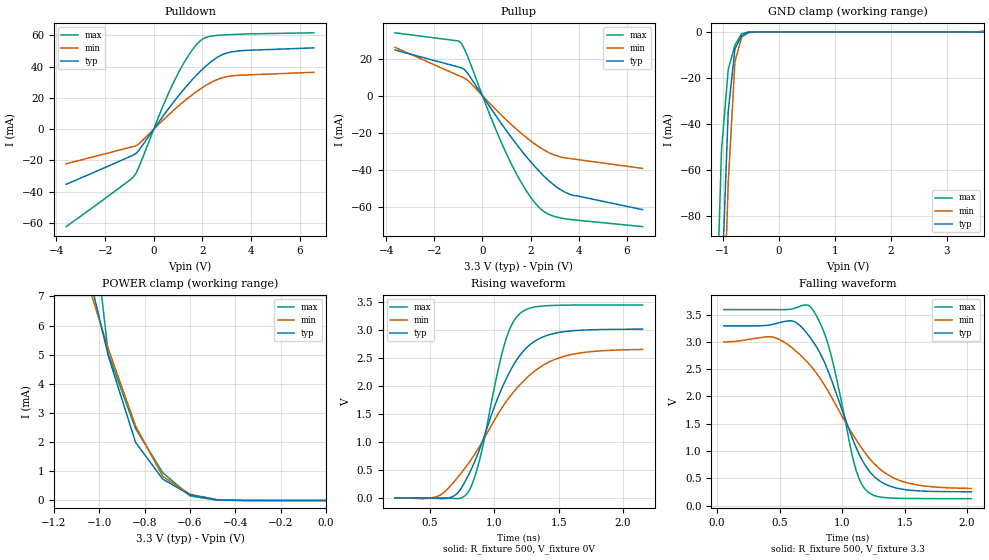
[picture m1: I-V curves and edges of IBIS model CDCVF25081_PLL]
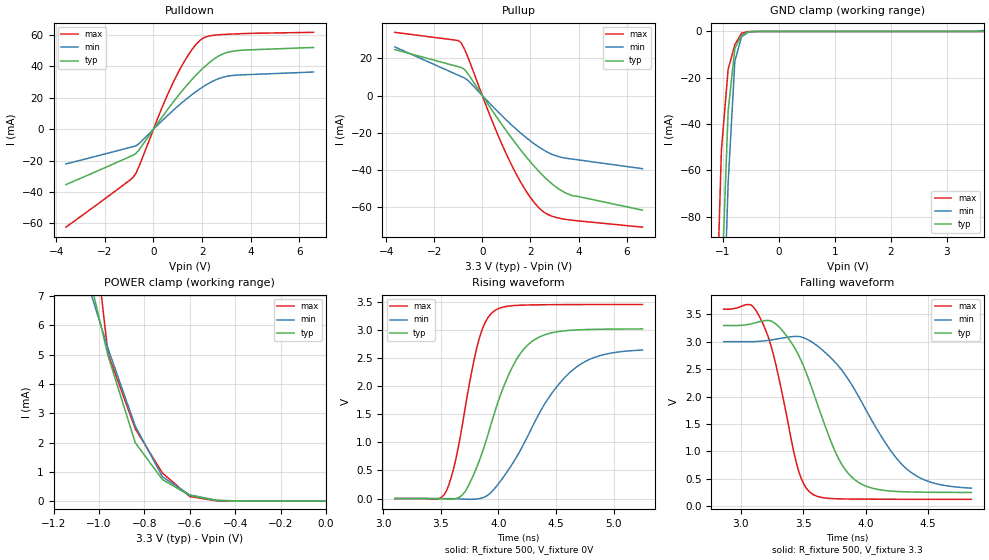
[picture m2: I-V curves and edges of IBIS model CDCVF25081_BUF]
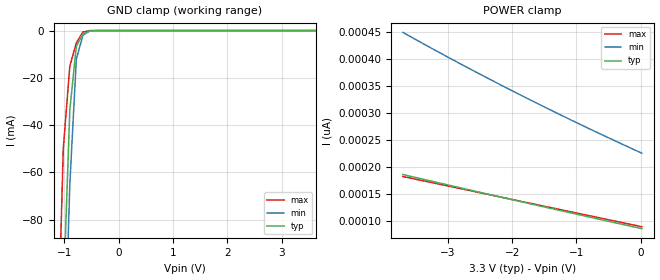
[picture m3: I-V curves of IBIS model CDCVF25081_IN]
[IBIS Ver]   3.2
[File Name]   cvf25081_03.ibs  | DEVICES: CDCVF25081PW
[File Rev]   0.3
[Date]   11/15/2002
[Source]   File originated at Texas Instruments
[Notes]   The following information corresponds to the
|   CDCVF25081 output buffers and input ESD circuits.
|Revision log: 0.1, 11/12/2002  initial release.
|   0.2, 11/15/2002  DC/AC correlation CDCVF25081
|   0.3, 11/22/2002  added model spec parameter
| Simulation hints.
| In PLL-MODE the Vt tables are normalized to have them switching all at the
| same time across TYP/MIN/MAX to reflect the virtual independency on split,
| VDD and temperature due to active phase controll in PLL-MODE.
| However there is a positive offset, since real phase relation in PLL_MODE
| would require negative relation to input signal which can not be simulated
| within IBIS models!
| In simple buffer mode the model works as a buffer and the VT plots represent
| the buffer switching characteristics starting at Vmeas for input signal, which
| initiates the buffer to toggle. If the lead-in delay is unwanted, equally
| substract exact same amount of time from rising AND falling waveforms !
[Disclaimer]
|This information is for modeling purposes only
|and is not guaranteed.
|Property of Texas Instruments Incorporated unauthorized reproduction
|and/or distribution is strictly prohibited.
|This product is protected under copyright law and trade
|secret law as an unpublished work.  Created  1998.
|(C) Copyright 1998 Texas Instruments Incorporated.
|All rights reserved.
|These commodities are under U.S. Government distribution
|license control. As such, they are not to be re-exported
|without prior approval of the U.S. Department of Commerce.
|Please be aware that in the absence of a written agreement
|to the contrary, Texas Instruments ("TI") assumes no
|liability for:  (1) the accuracy of the IBIS Models provided
|to your company;  (2) the proper functioning of these Models
|in your design system or for any resulting applications;
|or (3) infringement of patents, copyrights or intellectual
|property rights resulting from your use of these models.
|TI provides IBIS Models as a service to our customers
|and therefore reserves the right to limit distribution
|of the Models.
|CDCVF25081 IBIS I/O Model
|Mixed Signal Products, Texas Instruments
[Component]   CDCVF25081PW   | 16 Pin TSSOP package
[Manufacturer] Texas Instruments
[Package]
|   typ   min   max
R_pkg   0.0450710   0.0376501   0.0513656
L_pkg   2.5907775n   2.44687n   3.07983n
C_pkg   0.1415751p   0.0907328p   0.270926p
[Pin]   signal_name   model_name   R_pin   L_pin   C_pin
 1   CLK   CDCVF25081_IN   0.0397681   3.07983n   0.270926p
 2   1Y0   CDCVF25081_OUT   0.0376501   2.45757n   0.138771p
 3   1Y1   CDCVF25081_OUT   0.0512415   2.51196n   0.115722p
 4   VDD   POWER   0.0513168   2.44723n   0.090733p
 5   GND   GND   0.0513659   2.44724n   0.097386p
 6   2Y0   CDCVF25081_OUT   0.0512883   2.51196n   0.115722p
 7   2Y1   CDCVF25081_OUT   0.0376511   2.45777n   0.138759p
 8   S2   CDCVF25081_CTRLIN   0.0397673   3.03973n   0.270941p
 9   S1   CDCVF25081_CTRLIN   0.0394705   2.83153n   0.216335p
10   2Y2   CDCVF25081_OUT   0.0384835   2.45963n   0.142304p
11   2Y3   CDCVF25081_OUT   0.0512411   2.51159n   0.115740p
12   GND   GND   0.0513654   2.44687n   0.090831p
13   VDD   POWER   0.0513656   2.44687n   0.090825p
14   1Y2   CDCVF25081_OUT   0.0512413   2.51157n   0.115741p
15   1Y3   CDCVF25081_OUT   0.0384826   2.45948n   0.142306p
16   FBIN   CDCVF25081_IN   0.0394374   2.83161n   0.216310p
[Model Selector]   CDCVF25081_OUT
CDCVF25081_BUF for SIMPLE_BUFFER_MODE
CDCVF25081_PLL for PLL_MODE
| Models and submodels in the file (4): CDCVF25081_PLL (Output), CDCVF25081_BUF (Output), CDCVF25081_IN (Input), CDCVF25081_CTRLIN (Input)
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|   Model CDCVF25081_PLL
[Model]   CDCVF25081_PLL
Model_type   Output
Polarity   Non-Inverting
Enable   Active-High
Vmeas = 1.5V
Cref = 15pF
Rref = 500
Vref = 1.65V
|   variable   typ   min   max
C_comp   2.8pF   NA   NA
[Model Spec]
|  subparameter   typ   min   max
Vmeas   1.65V   1.50V   1.80V
|   variable   typ   min   max
[Temperature Range]   40   85   -40
[Voltage range]   3.3   3.0   3.6
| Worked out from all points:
|   slope of the pulldown table from 0 to 0.495 V, typ, clamps not added: 46.1 ohm
|   slope of the pullup table from 0 to 0.495 V, typ, clamps not added: 51.6 ohm
|   GND clamp passes 1 mA (typ) near -0.61 V on its own axis
|   POWER clamp passes 1 mA (typ) near -0.75 V on its own axis
|   rising waveform, R_fixture 500, V_fixture 0V: 20-80 % time 320ps typ, 470ps min, 194ps max; typ from 0 V to 3.02 V
|   falling waveform, R_fixture 500, V_fixture 3.3: 20-80 % time 307ps typ, 440ps min, 196ps max; typ from 3.3 V to 0.252 V
[Pullup]
|   40C:3.3V:nominal   85C:3.0V:weak   -40C:3.6V:strong
|  Voltage   I(typ)   I(min)   I(max)
-3.64V    24.7mA     26.12mA    33.95mA
-1V       15.51mA    10.93mA    29.56mA
-880mV    15.09mA    10.23mA    28.31mA
-640mV    12.45mA    8.62mA     21.96mA
440mV     -8.541mA   -5.947mA   -14.63mA
1.16V     -21.74mA   -15.05mA   -35.71mA
1.88V     -33.69mA   -23.11mA   -52.38mA
2.24V     -39.05mA   -26.59mA   -58.61mA
2.48V     -42.32mA   -28.63mA   -61.7mA
3.08V     -49.16mA   -32.29mA   -65.37mA
3.66V     -53.25mA   -33.88mA   -66.69mA
6.66V     -61.41mA   -39.18mA   -70.55mA
[Pulldown]
|   40C:3.3V:nominal   85C:3.0V:weak   -40C:3.6V:strong
|  Voltage   I(typ)   I(min)   I(max)
-3.6V     -35.29mA   -22.13mA   -62.34mA
-840mV    -16.57mA   -11.08mA   -30.65mA
-600mV    -13.26mA   -9.226mA   -23.82mA
340mV     7.461mA    5.189mA    13.35mA
820mV     17.44mA    12.14mA    30.1mA
1.3V      26.65mA    18.55mA    44.02mA
1.66V     32.94mA    22.91mA    52.28mA
1.9V      36.78mA    25.56mA    56.37mA
2.14V     40.29mA    27.97mA    58.65mA
2.62V     46.02mA    31.8mA     59.99mA
3.1V      49.13mA    33.84mA    60.45mA
6.58V     52.01mA    36.39mA    61.64mA
[GND Clamp]
|   40C:3.3V:nominal   85C:3.0V:weak   -40C:3.6V:strong
|  Voltage   I(typ)   I(min)   I(max)
-3.66V    -2.664A    -2.705A    -2.597A
-1.26V    -322.6mA   -368.2mA   -247.4mA
-1.02V    -113.4mA   -156.1mA   -51.21mA
-900mV    -34.44mA   -65.67mA   -16.35mA
-780mV    -7.275mA   -12.8mA    -5.698mA
-660mV    -1.683mA   -2.274mA   -709.9uA
-540mV    -157.1uA   -304.4uA   -20.32uA
-420mV    -6.863uA   -22.34uA   -162nA
3.42V     391.2pA    8.031uA    123.3pA
3.66V     873.2nA    432.9uA    136.7pA
[POWER Clamp]
|   40C:3.3V:nominal   85C:3.0V:weak  -40C:3.6V:strong
|  Voltage   I(typ)   I(min)   I(max)
-3.6V     107mA      79mA       290mA
-1.08V    8.909mA    8.202mA    13.19mA
-960mV    4.96mA     5.207mA    5.035mA
-840mV    1.996mA    2.561mA    2.466mA
-720mV    733.3uA    827.9uA    954.8uA
-600mV    191.2uA    212.2uA    157.3uA
-480mV    19.67uA    29.3uA     7.993uA
0V        126.6pA    280.9pA    133.2pA
[ramp]
| variable   typ   min   max
dV/dt_r   1.8115/3.2020E-10   1.5957/4.7143E-10   2.0668/1.9311E-10
dV/dt_f   1.8292/3.0774E-10   1.6162/4.4162E-10   2.0805/1.9637E-10
[Rising Waveform]
R_fixture = 500
V_fixture = 0V
|   40C:3.3V:nominal   85C:3.0V:weak   -40C:3.6V:strong
|   Time   V(typ)   V(min)   V(max)
231ps     0V         100uV      0V
570.5ps   -10.8mV    38.9mV     100uV
690.5ps   38.7mV     292.3mV    -9.4mV
790.5ps   363.5mV    585.1mV    75.9mV
890.5ps   889.4mV    936.1mV    708.3mV
1.091ns   2.116V     1.713V     2.828V
1.211ns   2.58V      2.048V     3.314V
1.351ns   2.846V     2.328V     3.422V
1.551ns   2.972V     2.534V     3.443V
2.151ns   3.015V     2.652V     3.447V
[Falling Waveform]
R_fixture = 500
V_fixture = 3.3
V_fixture_min = 3.0
V_fixture_max = 3.6
|   40C:3.3V:nominal   85C:3.0V:weak -40C:3.6V:strong
|   Time   V(typ)   V(min)   V(max)
54ps      3.296V     3.001V     3.593V
454ps     3.327V     3.085V     3.593V
614ps     3.377V     2.865V     3.613V
754ps     3.053V     2.549V     3.627V
894ps     2.432V     2.074V     2.912V
1.114ns   1.055V     1.202V     634mV
1.214ns   642.4mV    877.8mV    236mV
1.334ns   405.6mV    613.4mV    148.1mV
1.494ns   295.8mV    434.6mV    131.6mV
2.034ns   252.4mV    314.8mV    126.1mV
|   Model CDCVF25081_BUF
[Model]   CDCVF25081_BUF
Model_type   Output
Polarity   Non-Inverting
Enable   Active-High
Vmeas = 1.5V
Cref = 15pF
Rref = 500
Vref = 1.65V
|   variable   typ   min   max
C_comp   2.8pF   NA   NA
[Model Spec]
|  subparameter   typ   min   max
Vmeas   1.65V   1.50V   1.80V
|   variable   typ   min   max
[Temperature Range]   40   85   -40
[Voltage range]   3.3   3.0   3.6
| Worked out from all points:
|   slope of the pulldown table from 0 to 0.495 V, typ, clamps not added: 46.1 ohm
|   slope of the pullup table from 0 to 0.495 V, typ, clamps not added: 51.6 ohm
|   GND clamp passes 1 mA (typ) near -0.61 V on its own axis
|   POWER clamp passes 1 mA (typ) near -0.75 V on its own axis
|   rising waveform, R_fixture 500, V_fixture 0V: 20-80 % time 320ps typ, 466ps min, 194ps max; typ from 0 V to 3.02 V
|   falling waveform, R_fixture 500, V_fixture 3.3: 20-80 % time 307ps typ, 436ps min, 196ps max; typ from 3.3 V to 0.251 V
[Pullup]
|   40C:3.3V:nominal   85C:3.0V:weak   -40C:3.6V:strong
|  Voltage   I(typ)   I(min)   I(max)
-3.64V    24.7mA     26.12mA    33.95mA
-1V       15.51mA    10.93mA    29.56mA
-880mV    15.09mA    10.23mA    28.31mA
-640mV    12.45mA    8.62mA     21.96mA
440mV     -8.541mA   -5.947mA   -14.63mA
1.16V     -21.74mA   -15.05mA   -35.71mA
1.88V     -33.69mA   -23.11mA   -52.38mA
2.24V     -39.05mA   -26.59mA   -58.61mA
2.48V     -42.32mA   -28.63mA   -61.7mA
3.08V     -49.16mA   -32.29mA   -65.37mA
3.66V     -53.25mA   -33.88mA   -66.69mA
6.66V     -61.41mA   -39.18mA   -70.55mA
[Pulldown]
|   40C:3.3V:nominal   85C:3.0V:weak   -40C:3.6V:strong
|  Voltage   I(typ)   I(min)   I(max)
-3.6V     -35.29mA   -22.13mA   -62.34mA
-840mV    -16.57mA   -11.08mA   -30.65mA
-600mV    -13.26mA   -9.226mA   -23.82mA
340mV     7.461mA    5.189mA    13.35mA
820mV     17.44mA    12.14mA    30.1mA
1.3V      26.65mA    18.55mA    44.02mA
1.66V     32.94mA    22.91mA    52.28mA
1.9V      36.78mA    25.56mA    56.37mA
2.14V     40.29mA    27.97mA    58.65mA
2.62V     46.02mA    31.8mA     59.99mA
3.1V      49.13mA    33.84mA    60.45mA
6.58V     52.01mA    36.39mA    61.64mA
[GND Clamp]
|   40C:3.3V:nominal   85C:3.0V:weak   -40C:3.6V:strong
|  Voltage   I(typ)   I(min)   I(max)
-3.66V    -2.664A    -2.705A    -2.597A
-1.26V    -322.6mA   -368.2mA   -247.4mA
-1.02V    -113.4mA   -156.1mA   -51.21mA
-900mV    -34.44mA   -65.67mA   -16.35mA
-780mV    -7.275mA   -12.8mA    -5.698mA
-660mV    -1.683mA   -2.274mA   -709.9uA
-540mV    -157.1uA   -304.4uA   -20.32uA
-420mV    -6.863uA   -22.34uA   -162nA
3.42V     391.2pA    8.031uA    123.3pA
3.66V     873.2nA    432.9uA    136.7pA
[POWER Clamp]
|   40C:3.3V:nominal   85C:3.0V:weak  -40C:3.6V:strong
|  Voltage   I(typ)   I(min)   I(max)
-3.6V     107mA      79mA       290mA
-1.08V    8.909mA    8.202mA    13.19mA
-960mV    4.96mA     5.207mA    5.035mA
-840mV    1.996mA    2.561mA    2.466mA
-720mV    733.3uA    827.9uA    954.8uA
-600mV    191.2uA    212.2uA    157.3uA
-480mV    19.67uA    29.3uA     7.993uA
0V        126.6pA    280.9pA    133.2pA
[ramp]
| variable   typ   min   max
dV/dt_r   1.8115/3.2020E-10   1.5957/4.7143E-10   2.0668/1.9311E-10
dV/dt_f   1.8292/3.0774E-10   1.6162/4.4162E-10   2.0805/1.9637E-10
[Rising Waveform]
R_fixture = 500
V_fixture = 0V
|   40C:3.3V:nominal   85C:3.0V:weak   -40C:3.6V:strong
|   Time   V(typ)   V(min)   V(max)
3.1ns     0V         0V         0V
3.551ns   -10.8mV    100uV      146.4mV
3.631ns   500uV      -3.5mV     708.3mV
3.691ns   73.5mV     -8.9mV     1.365V
3.811ns   552.9mV    -8mV       2.67V
3.951ns   1.423V     140.4mV    3.314V
4.131ns   2.378V     649.5mV    3.431V
4.331ns   2.846V     1.424V     3.444V
4.711ns   3.001V     2.385V     3.449V
5.251ns   3.015V     2.64V      3.45V
[Falling Waveform]
R_fixture = 500
V_fixture = 3.3
V_fixture_min = 3.0
V_fixture_max = 3.6
|   40C:3.3V:nominal   85C:3.0V:weak -40C:3.6V:strong
|   Time   V(typ)   V(min)   V(max)
2.865ns   3.296V     3.001V     3.593V
3.085ns   3.326V     3.001V     3.669V
3.165ns   3.372V     3.01V      3.395V
3.265ns   3.352V     3.04V      2.741V
3.465ns   2.749V     3.095V     634mV
3.565ns   2.184V     3.001V     236mV
3.765ns   952.5mV    2.602V     136.1mV
3.945ns   431.7mV    1.995V     129.3mV
4.345ns   260.4mV    648.3mV    126.3mV
4.845ns   250.9mV    330mV      125.6mV
|   Model CDCVF25081_IN
[Model]   CDCVF25081_IN
Model_type   Input
Polarity   Non-Inverting
Vinl = 0.8V
Vinh = 2.0V
| variable   typ   min   max
C_comp   3.6pF   NA   NA
[Temperature Range]   40   85   -40
[Voltage range]   3.3   3.0   3.6
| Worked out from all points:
|   GND clamp passes 1 mA (typ) near -0.61 V on its own axis
|Process range   nominal   weak   strong
[GND Clamp]
|   40C:3.3V:nominal   85C:3.0V:weak  -40C:3.6V:strong
|  Voltage   I(typ)   I(min)   I(max)
-3.66V    -2.664A    -2.705A    -2.597A
-1.26V    -322.3mA   -368mA     -246.9mA
-1.02V    -112.9mA   -155.7mA   -49.9mA
-900mV    -33.58mA   -65.08mA   -15.03mA
-780mV    -6.672mA   -12.13mA   -5.186mA
-660mV    -1.52mA    -2.065mA   -636uA
-540mV    -141uA     -274.6uA   -17.91uA
-420mV    -6.132uA   -20.13uA   -140.8nA
3.64V     95.43pA    262.2pA    91.01pA
[POWER Clamp]
|   40C:3.3V:nominal   85C:3.0V:weak   -40C:3.6V:strong
|  Voltage   I(typ)   I(min)   I(max)
-3.7V     186.2pA    449.5pA    182.5pA
-2.74V    159.7pA    387.2pA    158.5pA
-1.78V    133.8pA    328.2pA    134.5pA
-940mV    111.3pA    279.1pA    113.5pA
20mV      85.94pA    225.8pA    89.51pA
